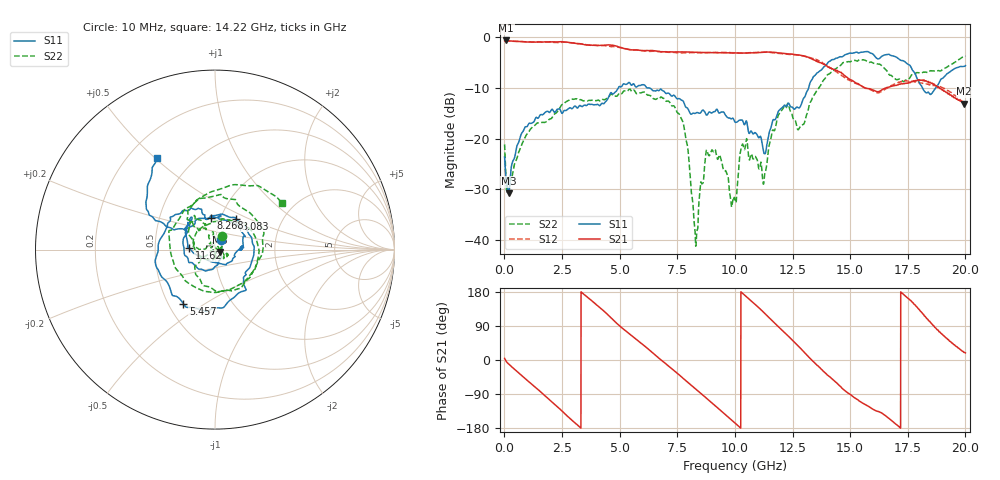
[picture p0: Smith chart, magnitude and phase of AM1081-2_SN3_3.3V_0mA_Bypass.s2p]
!Agilent Technologies,E8364B,MY43040894,A.07.50.67
!Agilent E8364B: A.07.50.67
!Date: Wednesday, June 23, 2021 08:06:04
!Correction: S11(Full 2 Port(1,2))
!S21(Full 2 Port(1,2))
!S12(Full 2 Port(1,2))
!S22(Full 2 Port(1,2))
!S2P File: Measurements: S11, S21, S12, S22:
# Hz S  dB  R 50
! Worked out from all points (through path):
!   3201 points, 10 MHz to 20 GHz, reference 50 ohm
!   highest |S21| = -0.61 dB at 72.47 MHz (marker M1); lowest = -13.1 dB at 19.95 GHz (marker M2)
!   group delay of S21, straight-line fit = 147 ps
!   lowest |S11| = -30.8 dB at 184.9 MHz (marker M3), VSWR 1.06, Z = 52.6 - j1.32 ohm
!   |S11| at or under -10 dB: start of sweep to 4.935 GHz; 6.289 GHz to 13.2 GHz (6.91 GHz wide, 70.9 % of centre); 18.14 GHz to 18.71 GHz (567.5 MHz wide, 3.08 % of centre)
!   |S22| runs from -41.3 to -3.7 dB; largest |S21 - S12| = 0.03
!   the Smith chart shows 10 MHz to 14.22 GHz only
!   S11 on the Smith chart (normalised r, x): 10 MHz: 1.07, +0.12; 3.083 GHz: 1.18, +0.43; 5.457 GHz: 0.60, -0.41; 8.268 GHz: 0.90, +0.33; 11.62 GHz: 0.75, +0.01; 14.22 GHz: 0.32, +0.51
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1e7  -23.64 57.5  -0.68 4.3  -0.65 3.6  -21.15 63.5
7.246875e7  -28.05 14.2  -0.61 -3.0  -0.64 -3.1  -29.22 12.8
1.849125e8  -30.83 -25.9  -0.70 -10.5  -0.72 -10.4  -27.96 -37.4
1.646681e9  -15.30 -179.5  -0.93 -88.1  -0.90 -88.6  -16.79 117.5
3.083462e9  -13.59 55.8  -1.17 -167.2  -1.15 -167.0  -12.14 -24.7
3.345831e9  -13.65 28.7  -1.28 178.6  -1.27 179.2  -12.38 -51.3
5.457275e9  -9.13 -120.2  -2.46 67.8  -2.39 68.0  -10.26 82.9
6.675416e9  -10.52 148.7  -2.77 5.8  -2.78 6.5  -12.14 -41.0
7.724891e9  -12.48 108.5  -2.88 -46.7  -3.07 -46.4  -16.48 -139.1
8.268369e9  -15.04 97.3  -2.95 -75.0  -3.00 -74.3  -38.08 -3.6
8.824341e9  -15.15 69.1  -2.99 -103.9  -3.01 -102.8  -22.94 -18.7
1.0005e10  -16.73 4.0  -3.07 -166.2  -3.03 -166.2  -32.07 162.0
1.161669e10  -16.83 176.6  -2.93 103.7  -3.04 103.6  -18.61 172.3
1.334083e10  -8.38 153.1  -4.26 -0.4  -4.15 0.4  -12.21 127.9
1.421539e10  -4.41 122.4  -6.24 -49.5  -6.22 -52.0  -6.86 35.0
1.547726e10  -2.95 42.0  -9.57 -111.3  -9.59 -110.5  -4.46 -66.7
1.667042e10  -3.34 -8.3  -9.85 -153.6  -9.84 -150.3  -7.23 -154.5
1.750125e10  -5.30 -42.7  -8.99 163.3  -8.60 160.5  -8.28 86.7
1.850075e10  -11.25 -156.7  -9.02 97.8  -9.48 100.8  -6.59 -10.2
1.925038e10  -7.08 129.4  -11.18 54.1  -10.55 54.4  -5.71 -97.6
1.995002e10  -5.73 92.7  -13.13 20.1  -13.00 17.2  -3.71 -169.2
2e10  -5.59 90.2  -13.04 18.7  -13.02 15.5  -3.73 -171.8
